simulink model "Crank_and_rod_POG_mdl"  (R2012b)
settings: Solver=ode45  StartTime=0.0  StopTime=10.0  RelTol=1e-3
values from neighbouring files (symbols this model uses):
  bm = 0*2*Nm/(100*rpm)    (= 0)    [Crank_and_rod_POG.m]
  bp = 0*5*N/(10*metri/sec)    (= 0)    [Crank_and_rod_POG.m]
  dot_H_th_out = subs(dot_H_th,th)    [Crank_and_rod_POG.m]
  Fp = 0*N    (= 0)    [Crank_and_rod_POG.m]
  H_th_out = subs(H_th,th)    [Crank_and_rod_POG.m]
  Jm = 500*gr*(5*cm)^2    (= 0.00125)    [Crank_and_rod_POG.m]
  mp = 800*gr    (= 0.8)    [Crank_and_rod_POG.m]
  Tc = Tfin/4000    (= 0.0005)    [Crank_and_rod_POG.m]
  Th_in = th    [Crank_and_rod_POG.m]
  Thm_0 = 0*rad    (= 0)    [Crank_and_rod_POG.m]
  Tm = 0*2*Nm    (= 0)    [Crank_and_rod_POG.m]
  Wm_0 = 200*rpm    (= 20.9439510239)    [Crank_and_rod_POG.m]

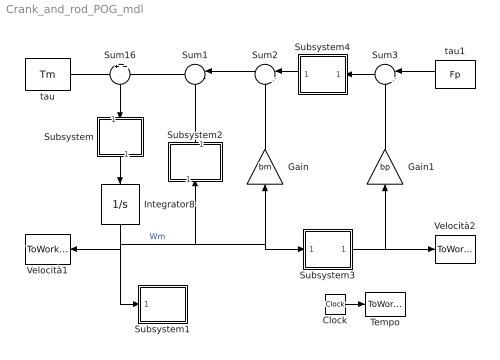
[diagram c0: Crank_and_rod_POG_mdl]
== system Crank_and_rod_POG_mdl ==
  Clock : Clock
  Gain : Gain  Gain=bm
  Gain1 : Gain  Gain=bp
  Integrator8 : Integrator  InitialCondition=Wm_0  LowerSaturationLimit=0
  Subsystem : Subsystem
  Subsystem1 : Subsystem
  Subsystem2 : Subsystem
  Subsystem3 : Subsystem
  Subsystem4 : Subsystem
  Sum1 : Sum  Inputs=|--
  Sum16 : Sum  Inputs=+|+
  Sum2 : Sum  Inputs=|++
  Sum3 : Sum  Inputs=|++
  Tempo : ToWorkspace  VariableName=t  SampleTime=Tc
  Velocità1 : ToWorkspace  VariableName=Wm  SampleTime=Tc
  Velocità2 : ToWorkspace  VariableName=dot_x  SampleTime=Tc
  tau : Constant  Value=Tm
  tau1 : Constant  Value=Fp
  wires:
  Clock/1 -> Tempo/1
  Integrator8/1 -> Velocità1/1, Subsystem2/1(Wm), Gain/1, Subsystem3/1(In), Subsystem1/1(In1)  "Wm"
  Sum1/1 -> Sum16/2
  Subsystem2/1(N1) -> Sum1/2
  tau/1 -> Sum16/1
  Gain/1 -> Sum2/2
  Sum2/1 -> Sum1/1
  Subsystem4/1(Out) -> Sum2/1
  Subsystem3/1(Out) -> Velocità2/1, Gain1/1
  Gain1/1 -> Sum3/2
  Sum3/1 -> Subsystem4/1(In)
  tau1/1 -> Sum3/1
  Sum16/1 -> Subsystem/1(In1)
  Subsystem/1(Out1) -> Integrator8/1

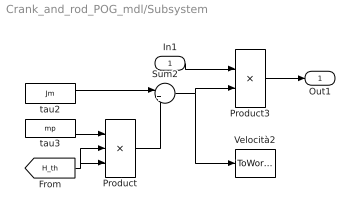
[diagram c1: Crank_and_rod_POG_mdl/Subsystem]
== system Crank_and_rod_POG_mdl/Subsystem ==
  In1 : Inport
  Product : Product  Inputs=3
  Product3 : Product  Inputs=*/
  Sum2 : Sum  Inputs=|++
  Velocità2 : ToWorkspace  VariableName=J_th  SampleTime=Tc
  tau2 : Constant  Value=Jm
  tau3 : Constant  Value=mp
  Out1 : Outport
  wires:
  tau3/1 -> Product/1
  [H_th] -> Product/2, Product/3
  tau2/1 -> Sum2/1
  Product/1 -> Sum2/2
  Sum2/1 -> Product3/2, Velocità2/1
  In1/1 -> Product3/1
  Product3/1 -> Out1/1

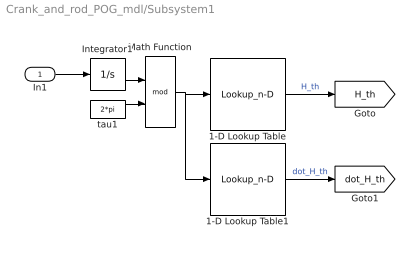
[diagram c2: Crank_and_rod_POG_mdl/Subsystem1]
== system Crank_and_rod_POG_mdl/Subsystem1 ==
  In1 : Inport
  1-D Lookup Table : Lookup_n-D  NumberOfTableDimensions=1  BreakpointsForDimension1=Th_in  Table=H_th_out  RndMeth=Simplest
  1-D Lookup Table1 : Lookup_n-D  NumberOfTableDimensions=1  BreakpointsForDimension1=Th_in  Table=dot_H_th_out  RndMeth=Simplest
  Integrator1 : Integrator  InitialCondition=Thm_0  LowerSaturationLimit=0
  Math Function : Math  Operator=mod
  tau1 : Constant  Value=2*pi
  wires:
  Integrator1/1 -> Math Function/1
  tau1/1 -> Math Function/2
  Math Function/1 -> 1-D Lookup Table/1, 1-D Lookup Table1/1
  1-D Lookup Table/1 -> [H_th]  "H_th"
  1-D Lookup Table1/1 -> [dot_H_th]  "dot_H_th"
  In1/1 -> Integrator1/1

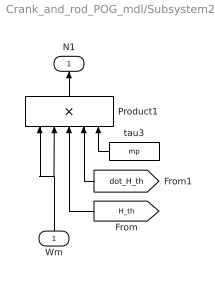
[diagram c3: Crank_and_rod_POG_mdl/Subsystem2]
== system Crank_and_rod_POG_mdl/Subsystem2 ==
  Wm : Inport
  Product1 : Product  Inputs=5
  tau3 : Constant  Value=mp
  N1 : Outport
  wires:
  [H_th] -> Product1/3
  [dot_H_th] -> Product1/4
  tau3/1 -> Product1/5
  Wm/1 -> Product1/1, Product1/2
  Product1/1 -> N1/1

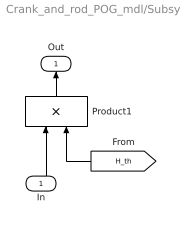
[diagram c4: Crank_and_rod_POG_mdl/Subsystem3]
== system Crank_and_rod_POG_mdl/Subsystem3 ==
  In : Inport
  Product1 : Product
  Out : Outport
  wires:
  Product1/1 -> Out/1
  In/1 -> Product1/1
  [H_th] -> Product1/2

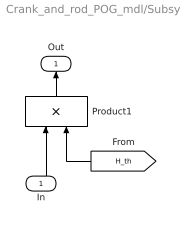
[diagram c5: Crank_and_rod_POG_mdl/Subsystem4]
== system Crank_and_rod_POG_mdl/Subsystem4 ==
  In : Inport
  Product1 : Product
  Out : Outport
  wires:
  [H_th] -> Product1/2
  In/1 -> Product1/1
  Product1/1 -> Out/1
